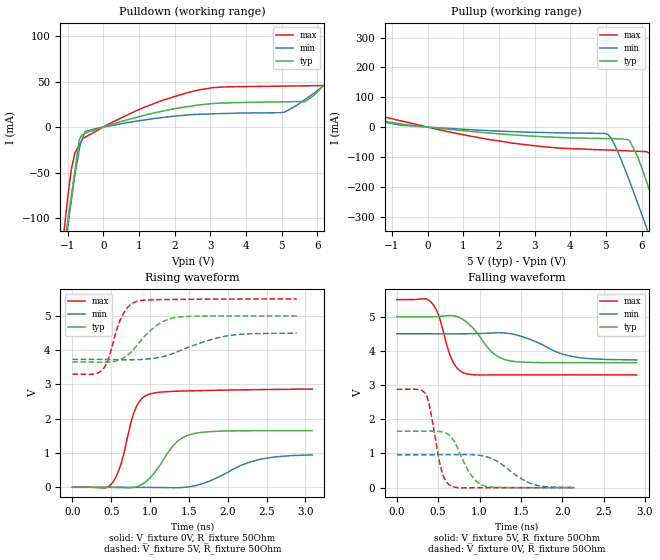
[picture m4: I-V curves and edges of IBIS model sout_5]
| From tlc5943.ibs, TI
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|   sout_5 Model
[Model]   sout_5
Model_type   Output
Polarity   Non-Inverting
Vmeas = 2.5
Vref = 2.5
Cref = 15pF
Rref = 50
|   typ   min   max
|   (nom PVT)   (Fast PVT)   (slow PVT)
|Average
C_comp   1.688e-12   1.601e-12   1.694e-12
|ON state : BUFFER OUTPUT TURNED HIGH
|C_comp   1.688e-12   1.601e-12   1.694e-12
|OFF state: BUFFER OUTPUT TURNED LOW
|C_comp   1.453e-12   1.437e-12   1.473e-12
| Where nom  PVT is Nominal Process,  5V,  65C
|   Fast PVT is Strong Process,   5.5V,  -40C
|   Slow PVT is Weak Process,   4.5V,  125C
[Voltage Range]   5   4.5   5.5
|Ambient Temperature   25   85   -40
|Junction Temperature
[Temperature Range]   65   125   -40
[Pullup Reference]   5   4.5   5.5
[Pulldown Reference]   0   0   0
[Power Clamp Reference]   5   4.5   5.5
[GND Clamp Reference]   0   0   0
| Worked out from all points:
|   slope of the pulldown table from 0 to 0.75 V, typ, clamps not added: 85.7 ohm
|   slope of the pullup table from 0 to 0.75 V, typ, clamps not added: 81.5 ohm
|   falling waveform, V_fixture 5V, R_fixture 50Ohm: 20-80 % time 274ps typ, 433ps min, 164ps max; typ from 5 V to 3.66 V
|   rising waveform, V_fixture 0V, R_fixture 50Ohm: 20-80 % time 322ps typ, 544ps min, 203ps max; typ from 0 V to 1.65 V
|   rising waveform, V_fixture 5V, R_fixture 50Ohm: 20-80 % time 343ps typ, 572ps min, 193ps max; typ from 3.65 V to 5 V
|   falling waveform, V_fixture 0V, R_fixture 50Ohm: 20-80 % time 208ps typ, 339ps min, 131ps max; typ from 1.65 V to 0 V
[Pulldown]
|   Voltage   I(typ)   I(min)   I(max)
-5V       -1.696A    -1.53A     -1.982A
-1.117V   -136.5mA   -146.4mA   -120.9mA
-1.001V   -104.7mA   -111.2mA   -79.43mA
-797.5mV  -48.83mA   -53.36mA   -28.91mA
-670mV    -13.8mA    -24.04mA   -19.72mA
-499.5mV  -6.814mA   -4.765mA   -10.99mA
2.376V    22.54mA    13.36mA    38mA
5.076V    27.76mA    16.27mA    45.07mA
6.353V    53.33mA    50.33mA    45.85mA
6.886V    76.57mA    65.9mA     85.77mA
8.52V     151mA      116.2mA    235mA
10V       224.1mA    161.8mA    381.2mA
[Pullup]
|   Voltage   I(typ)   I(min)   I(max)
-5V       186.1mA    126.6mA    362.9mA
-4.5V     163.9mA    112mA      318.2mA
-1.188V   20.02mA    15.84mA    33.16mA
2.36V     -25.82mA   -15.23mA   -53.37mA
4.959V    -38.48mA   -21.29mA   -76.65mA
5.252V    -39.18mA   -60.95mA   -77.79mA
5.66V     -44.8mA    -180.6mA   -79.92mA
6.138V    -181.6mA   -336.9mA   -82.41mA
6.407V    -279.2mA   -430.4mA   -114.4mA
6.578V    -343mA     -489.6mA   -179.6mA
6.891V    -463.8mA   -598.9mA   -318.5mA
10V       -1.741A    -1.738A    -1.821A
[Ramp]
R_load = 50
|   typ   min   max
dV/dt_r   0.990386/3.21505e-10   0.574441/5.52625e-10   1.72204/2.03389e-10
dV/dt_f   0.806694/2.73235e-10   0.461239/4.34455e-10   1.31991/1.63927e-10
[Falling Waveform]
V_fixture = 5V
V_fixture_min = 4.5V
V_fixture_max = 5.5V
R_fixture = 50Ohm
|   Time   V(typ)   V(min)   V(max)
0s        5V         4.5V       5.5V
350ps     4.999V     4.5V       5.522V
420ps     5.001V     4.5V       5.41V
500ps     5.008V     4.5V       5.082V
670ps     5.03V      4.499V     3.725V
830ps     4.869V     4.501V     3.339V
1.13ns    4.012V     4.521V     3.298V
1.33ns    3.73V      4.519V     3.3V
2.06ns    3.656V     3.868V     3.3V
2.9ns     3.656V     3.735V     3.3V
[Rising Waveform]
V_fixture = 0V
V_fixture_min = 0V
V_fixture_max = 0V
R_fixture = 50Ohm
|   Time   V(typ)   V(min)   V(max)
0s        305.8pV    1.76nV     264.4pV
430ps     -926uV     464.3uV    -16.25mV
510ps     -3.884mV   668.9uV    118.4mV
630ps     -10.38mV   626.6uV    719.9mV
810ps     7.526mV    -1.02mV    2.284V
970ps     212.4mV    -3.629mV   2.7V
1.31ns    1.246V     -14.33mV   2.8V
1.5ns     1.525V     13.33mV    2.814V
2.38ns    1.65V      795.8mV    2.848V
3.09ns    1.651V     946.3mV    2.865V
[Rising Waveform]
V_fixture = 5V
V_fixture_min = 4.5V
V_fixture_max = 5.5V
R_fixture = 50Ohm
|   Time   V(typ)   V(min)   V(max)
0s        3.655V     3.731V     3.3V
280ps     3.651V     3.731V     3.304V
390ps     3.645V     3.729V     3.441V
460ps     3.65V      3.727V     3.733V
640ps     3.75V      3.72V      4.998V
840ps     4.168V     3.724V     5.433V
1.09ns    4.73V      3.779V     5.473V
1.33ns    4.957V     3.933V     5.481V
2.04ns    4.999V     4.433V     5.492V
2.89ns    5V         4.496V     5.497V
[Falling Waveform]
V_fixture = 0V
V_fixture_min = 0V
V_fixture_max = 0V
R_fixture = 50Ohm
|   Time   V(typ)   V(min)   V(max)
0s        1.651V     961.7mV    2.877V
350ps     1.653V     961.5mV    2.743V
400ps     1.654V     961.7mV    2.332V
540ps     1.634V     963.1mV    516.9mV
580ps     1.608V     963.6mV    252.2mV
660ps     1.471V     965.1mV    45.91mV
890ps     398.2mV    964.2mV    -2.71mV
1.05ns    57.68mV    922.7mV    87.85uV
1.66ns    377.8uV    90.52mV    340.8uV
2.15ns    151.3uV    4.467mV    333.7uV
